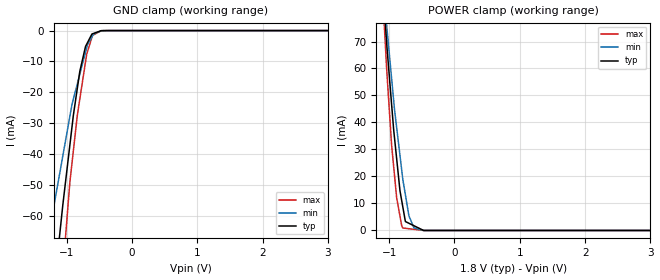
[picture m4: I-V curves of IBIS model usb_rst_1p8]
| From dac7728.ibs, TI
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|   usb_rst_1p8 Model
[Model]   usb_rst_1p8
Model_type   Input
Vinl = 0.3
Vinh = 1.5
|   typ   min   max
|   (nom PVT)   (Fast PVT)   (slow PVT)
|C_comp from frequency method(F=50MHz)
|Average
|C_comp   1.058e-11   8.952e-12   1.206e-11
|C_comp from L-C Tank method(L=1nH)
|Resonant Frequency(Hz)   1.61e9   1.73e9   1.52e9
C_comp   9.782e-12   8.472e-12   1.097e-11
| Where nom  PVT is Nominal Process,  1.8V,  33C
|   Fast PVT is Strong Process,   1.89V,  -40C
|   Slow PVT is Weak Process,   1.71V,  113C
[Voltage Range]   1.8   1.71   1.89
|Ambient Temperature   25   105   -40
|Junction Temperature
[Temperature Range]   33   113   -40
[Power Clamp Reference]   1.8   1.71   1.89
[GND Clamp Reference]   0   0   0
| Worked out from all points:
|   GND clamp passes 1 mA (typ) near -0.60 V on its own axis
|   POWER clamp passes 1 mA (typ) near -0.56 V on its own axis
[GND Clamp]
|   Voltage   I(typ)   I(min)   I(max)
-1.8V     -217.1mA   -140.2mA   -312.5mA
-1.262V   -97.62mA   -64.76mA   -140mA
-1.217V   -88.59mA   -59.47mA   -125.7mA
-1.058V   -56.53mA   -40.62mA   -77.97mA
-952.6mV  -37.5mA    -28.06mA   -49.75mA
-916.6mV  -31.03mA   -23.81mA   -42.75mA
-835.4mV  -18.63mA   -17.2mA    -27.34mA
-797.4mV  -13.17mA   -14.11mA   -22.1mA
-693.6mV  -4.462mA   -5.652mA   -7.799mA
-612mV    -1.105mA   -2.018mA   -2.18mA
-447.9mV  -29.85uA   -62.66uA   -17.6uA
3.6V      0A         0A         0A
[POWER Clamp]
|   Voltage   I(typ)   I(min)   I(max)
-1.8V     358mA      304.5mA    426.4mA
-1.132V   102.5mA    100.6mA    102.4mA
-1.033V   68.07mA    74.92mA    58.33mA
-960.1mV  46.27mA    55.98mA    31.26mA
-884.5mV  26.67mA    38.19mA    12.16mA
-833.4mV  14.7mA     27.77mA    5.309mA
-790mV    8.732mA    18.93mA    916.8uA
-750.6mV  3.31mA     13.22mA    803.6uA
-696mV    2.662mA    5.386mA    646.8uA
-619mV    1.749mA    918.7uA    426uA
-470.3mV  197.2nA    12.34uA    3.023nA
3.6V      0A         0A         0A
